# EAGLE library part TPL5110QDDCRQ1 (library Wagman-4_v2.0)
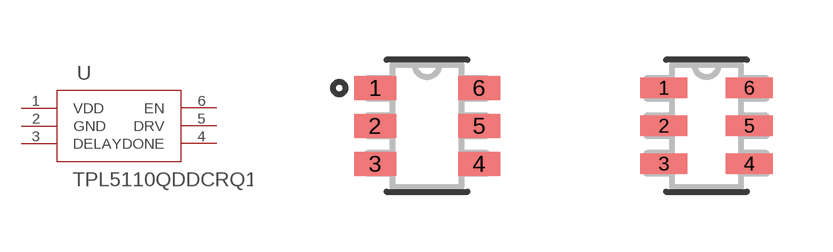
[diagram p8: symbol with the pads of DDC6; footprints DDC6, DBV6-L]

Designator prefix U

## TPL5110QDDCRQ1 (MANUFACTURER_PART_NUMBER: TPS3808G50DBVR; VENDOR: Texas Instruments)  [DDC6]
1  VDD  pas
2  GND  pwr
3  DELAY  pas
4  DONE  pas
5  DRV  pas
6  EN  pwr

## TPL5110QDDCRQ1DBV6-L (MANUFACTURER_PART_NUMBER: TPS3808G50DBVR; VENDOR: Texas Instruments)  [DBV6-L]
Pads as for DDC6

## TPL5110QDDCRQ1DBV6-M (MANUFACTURER_PART_NUMBER: TPS3808G50DBVR; VENDOR: Texas Instruments)  [DBV6-M]
Pads as for DDC6

## Footprint DDC6 (pad centres in mm)
smd 1.05 x 0.6: 1 -1.3,0.95; 2 -1.3,0; 3 -1.3,-0.95; 4 1.3,-0.95; 5 1.3,0; 6 1.3,0.95

## Footprint DBV6-L (pad centres in mm)
smd 1.168 x 0.508: 1 -1.067,0.95; 2 -1.067,0; 3 -1.067,-0.95; 4 1.067,-0.95; 5 1.067,0; 6 1.067,0.95

## Footprint DBV6-M (pad centres in mm)
smd 1.778 x 0.61: 1 -1.168,0.95; 2 -1.168,0; 3 -1.168,-0.95; 4 1.168,-0.95; 5 1.168,0; 6 1.168,0.95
